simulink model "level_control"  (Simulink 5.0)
settings: Solver=ode45  StartTime=0.0  StopTime=50  RelTol=1e-6
libraries: simulink x1

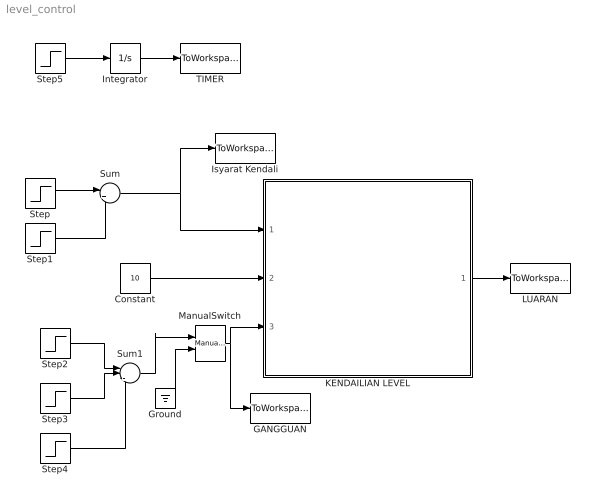
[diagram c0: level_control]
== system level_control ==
  Constant : Constant  Value=10
  GANGGUAN : ToWorkspace  VariableName=gangguan  SampleTime=-1  SaveFormat=Array
  Ground : Ground
  Integrator : Integrator
  Isyarat Kendali : ToWorkspace  VariableName=pompa  SampleTime=-1  SaveFormat=Array
  KENDAILIAN LEVEL : Subsystem
  LUARAN : ToWorkspace  VariableName=level  SampleTime=-1  SaveFormat=Array
  ManualSwitch : simulink/Signal Routing/Manual Switch  sw=1  action=0
  Step : Step  Time=5  After=40  SampleTime=0
  Step1 : Step  Time=17  After=35  SampleTime=0
  Step2 : Step  Time=9  After=10  SampleTime=0
  Step3 : Step  Time=12  SampleTime=0
  Step4 : Step  Time=14  SampleTime=0
  Step5 : Step  Time=0  SampleTime=0
  Sum : Sum  Inputs=|+-
  Sum1 : Sum  Inputs=|+--
  TIMER : ToWorkspace  VariableName=time  SampleTime=-1  SaveFormat=Array
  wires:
  Constant/1 -> KENDAILIAN LEVEL/2(KATUP manual)
  Step/1 -> Sum/1
  Step1/1 -> Sum/2
  Sum/1 -> KENDAILIAN LEVEL/1(pengendali POMPA), Isyarat Kendali/1
  Step2/1 -> Sum1/1
  Step3/1 -> Sum1/2
  Step4/1 -> Sum1/3
  KENDAILIAN LEVEL/1(level) -> LUARAN/1
  Step5/1 -> Integrator/1
  Integrator/1 -> TIMER/1
  ManualSwitch/1 -> KENDAILIAN LEVEL/3(KATUP otomatis), GANGGUAN/1
  Sum1/1 -> ManualSwitch/1
  Ground/1 -> ManualSwitch/2

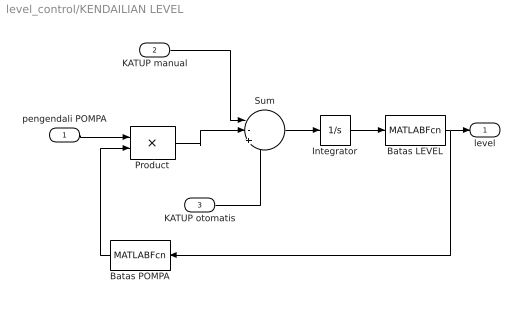
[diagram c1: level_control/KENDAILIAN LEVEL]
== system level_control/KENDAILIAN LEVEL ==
  pengendali POMPA : Inport
  KATUP manual : Inport  Port=2
  KATUP otomatis : Inport  Port=3
  Batas LEVEL : MATLABFcn  MATLABFcn=batas_level
  Batas POMPA : MATLABFcn  Orientation=left  MATLABFcn=batas_pompa
  Integrator : Integrator  InitialCondition=200
  Product : Product
  Sum : Sum  Inputs=|-+-
  level : Outport
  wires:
  Batas LEVEL/1 -> level/1, Batas POMPA/1
  Integrator/1 -> Batas LEVEL/1
  Sum/1 -> Integrator/1
  KATUP manual/1 -> Sum/1
  KATUP otomatis/1 -> Sum/3
  pengendali POMPA/1 -> Product/1
  Batas POMPA/1 -> Product/2
  Product/1 -> Sum/2
